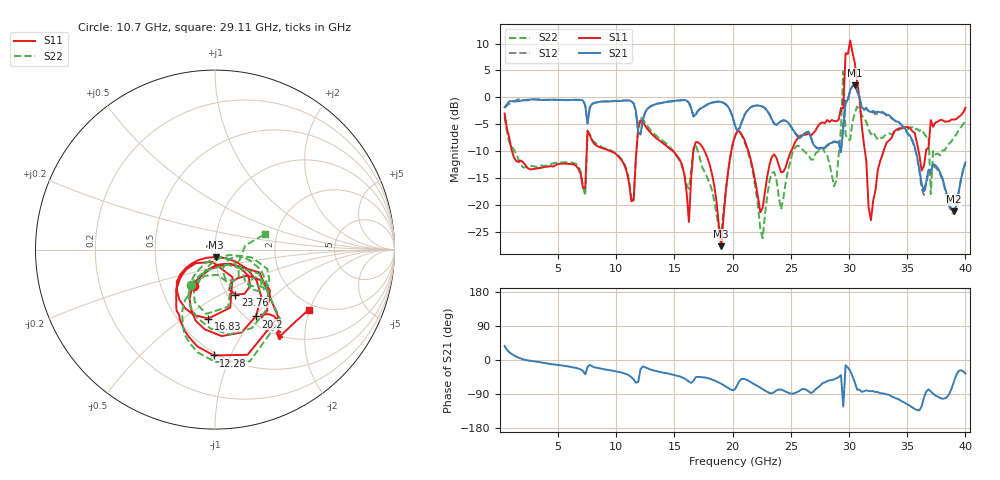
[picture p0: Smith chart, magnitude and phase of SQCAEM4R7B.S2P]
! Network Analyzer HP8722ES.07.66: Jul 25, 2000 Serial No. US39175408
! 26 Oct 2004  14:29:16
! Frequency  S11  S21  S12  S22
# HZ  S  DB R  50
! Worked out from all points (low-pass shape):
!   201 points, 400 MHz to 40 GHz, reference 50 ohm
!   highest |S21| = 2.25 dB at 30.5 GHz (marker M1); lowest = -21.2 dB at 39.01 GHz (marker M2)
!   |S21| within 3 dB of the highest: 780.7 MHz to 7.173 GHz (6.393 GHz wide, 161 % of centre); 9.061 GHz to 11.3 GHz (2.242 GHz wide, 22 % of centre)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
!   lowest |S11| = -27.6 dB at 19.01 GHz (marker M3), VSWR 1.09, Z = 50.4 - j4.17 ohm
!   |S11| at or under -10 dB: 1.046 GHz to 7.456 GHz (6.411 GHz wide, 151 % of centre); 17.59 GHz to 19.88 GHz (2.281 GHz wide, 12.2 % of centre); 21.36 GHz to 25.01 GHz (3.658 GHz wide, 15.8 % of centre)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
!   |S22| runs from -26.1 to 4.8 dB; largest |S21 - S12| = 0.12
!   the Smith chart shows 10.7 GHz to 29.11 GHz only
!   S11 on the Smith chart (normalised r, x): 10.7 GHz: 0.73, -0.31; 12.28 GHz: 0.48, -0.87; 16.83 GHz: 0.70, -0.63; 20.2 GHz: 1.10, -1.01; 23.76 GHz: 1.09, -0.59; 29.11 GHz: 1.81, -1.97
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4e8  -2.99 -54.8  -1.83 37.2  -1.93 41.6  -3.67 -46.8
7.132e9  -16.75 -102.3  -0.56 -28.9  -0.55 -29.3  -16.44 -113.8
1.0696e10  -12.58 -120.3  -0.58 -35.5  -0.56 -35.6  -12.35 -124.3
1.228e10  -4.59 -90.7  -4.15 -16.8  -4.10 -16.8  -4.06 -89.8
1.3666e10  -7.89 -122.0  -1.11 -31.0  -1.10 -31.1  -7.56 -115.8
1.624e10  -23.10 -102.2  -0.96 -57.2  -0.96 -57.3  -16.98 -84.3
1.6834e10  -8.27 -95.5  -3.16 -45.2  -3.17 -45.5  -8.84 -97.7
1.9012e10  -27.60 -81.7  -0.85 -62.5  -0.88 -62.8  -25.05 -46.1
2.02e10  -7.20 -58.6  -5.25 -77.3  -5.20 -76.7  -7.11 -49.1
2.3764e10  -11.20 -65.6  -5.09 -80.0  -5.11 -80.3  -15.32 -70.6
2.6932e10  -6.61 -50.3  -8.72 -83.7  -8.71 -83.7  -11.50 -34.9
2.911e10  -4.14 -32.5  -8.21 -45.2  -8.34 -45.2  -10.73 17.1
2.9506e10  -2.03 13.1  -5.57 -122.9  -4.86 -111.4  4.81 53.6
2.9704e10  8.21 1.1  -1.11 -13.9  -0.63 -7.4  -6.91 -70.0
3.01e10  10.57 -83.2  1.39 -28.2  1.31 -29.5  -7.85 0.7
3.0496e10  6.41 -115.5  2.25 -58.6  2.15 -58.4  -2.89 -24.1
3.0694e10  3.00 32.8  1.11 -78.1  1.19 -77.9  -1.70 139.6
3.1288e10  -8.78 1.9  -2.17 -82.7  -2.34 -83.6  -3.94 122.3
3.1486e10  -11.86 -144.7  -1.94 -80.0  -2.12 -81.2  -4.46 -60.1
3.3466e10  -7.94 -17.0  -3.32 -92.0  -3.59 -93.3  -6.66 -40.1
3.901e10  -4.12 -39.6  -21.16 -57.6  -21.61 -54.4  -7.36 27.1
4e10  -1.93 -30.8  -12.07 -35.8  -12.29 -33.9  -4.36 24.7
